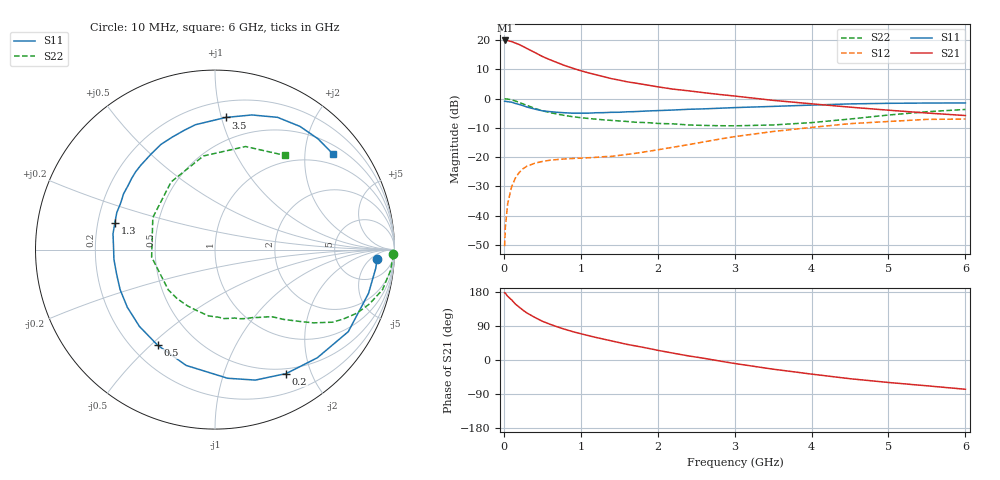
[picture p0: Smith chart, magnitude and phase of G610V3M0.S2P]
! SIEMENS Small Signal Semiconductors
! BFG193
! Si NPN RF Bipolar Junction Transistor in SOT223
! VCE = 10 V  IC = 3 mA
! Common Emitter S-Parameters:  August  1996
# GHz  S  MA  R  50
!  f  S11  S21  S12  S22
! GHz  MAG  ANG  MAG  ANG  MAG  ANG  MAG  ANG
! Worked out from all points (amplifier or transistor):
!   36 points, 10 MHz to 6 GHz, reference 50 ohm
!   highest |S21| = 19.9 dB at 20 MHz (marker M1)
!   |S21| within 3 dB of that: start of sweep to 318.8 MHz
!   unconditionally stable (mu >= 1): 1.3 GHz to 2.532 GHz
!   at 250 MHz: K = 0.22, MSG = 20.9 dB, |S12| = -24.0 dB
!   at 1.4 GHz: K = 1.06, MAG = 11.8 dB, |S12| = -19.7 dB
!   at 6 GHz: K = 0.90, MSG = 0.6 dB, |S12| = -7.0 dB
!   S11 on the Smith chart (normalised r, x): 10 MHz: 15, -8; 200 MHz: 0.44, -1.64; 500 MHz: 0.30, -0.53; 1.3 GHz: 0.27, +0.12; 3.5 GHz: 0.32, +1.03; 6 GHz: 0.71, +2.66
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0.01  0.9035 -3.2  9.881 177.5  0.003 90.7  0.9942 -1.5
0.02  0.9019 -6.5  9.92 176.2  0.0064 88.1  0.9916 -2.7
0.05  0.8894 -15.9  9.852 168.1  0.016 81.1  0.9842 -7.0
0.1  0.8721 -31.6  9.487 158.9  0.0308 73.4  0.9594 -13.5
0.15  0.8296 -46.6  8.949 147.7  0.044 64.8  0.9122 -19.4
0.2  0.7965 -60.1  8.44 139.5  0.0547 58.8  0.8666 -24.1
0.25  0.761 -72.8  7.829 131.3  0.0634 53.3  0.8131 -28.4
0.3  0.7203 -84.4  7.229 124.1  0.07 48.5  0.7696 -31.7
0.4  0.665 -104.0  6.198 112.7  0.0785 41.3  0.6846 -36.6
0.5  0.6211 -121.0  5.283 102.3  0.0844 36.1  0.6221 -40.1
0.6  0.6004 -134.5  4.641 94.4  0.0887 32.8  0.5789 -42.9
0.7  0.5847 -146.7  4.116 87.1  0.0911 30.5  0.544 -45.6
0.8  0.5737 -157.2  3.657 80.6  0.0934 29.1  0.5139 -47.7
1.1  0.5657 178.2  2.768 64.3  0.0976 28.9  0.4588 -55.2
1.3  0.5775 165.1  2.377 54.9  0.102 30.0  0.4344 -60.5
1.6  0.5968 148.6  1.949 41.3  0.1113 32.5  0.4081 -70.7
2.2  0.6399 124.0  1.458 18.1  0.148 34.8  0.3714 -95.4
2.8  0.6866 104.4  1.183 -2.5  0.2034 29.8  0.3452 -127.5
3.5  0.7385 85.4  0.937 -24.2  0.2748 16.1  0.3555 -173.3
4.5  0.8151 64.7  0.717 -49.4  0.3745 -6.2  0.4493 123.0
5.5  0.8429 47.1  0.569 -68.1  0.443 -34.4  0.599 73.5
6  0.8463 38.9  0.515 -77.2  0.4486 -49.9  0.6548 53.2
